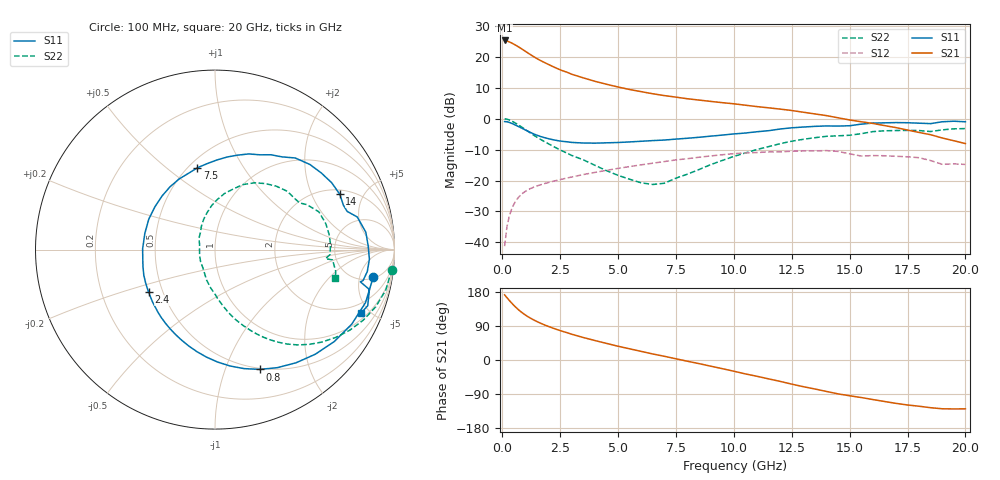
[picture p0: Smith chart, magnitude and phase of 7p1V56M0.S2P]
! Infineon Technologies  Discrete & RF Semiconductors
! bfp620
! VCE =  1.5 V,  IC =  6.0 mA
! Common Emitter S-Parameters:  Sep 2002
# GHz  S  MA  R  50
!  f  S11  S21  S12  S22
! GHz  MAG  ANG  MAG  ANG  MAG  ANG  MAG  ANG
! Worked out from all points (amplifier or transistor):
!   59 points, 100 MHz to 20 GHz, reference 50 ohm
!   highest |S21| = 25.2 dB at 100 MHz (marker M1)
!   |S21| within 3 dB of that: start of sweep to 895 MHz
!   unconditionally stable (mu >= 1): 4.674 GHz to 11.28 GHz; 14.93 GHz to 15.1 GHz; 17.11 GHz to end of sweep
!   at 1 GHz: K = 0.36, MSG = 22.6 dB, |S12| = -23.5 dB
!   at 5.5 GHz: K = 1.04, MAG = 11.2 dB, |S12| = -15.5 dB
!   at 20 GHz: K = 1.39, MAG = -0.3 dB, |S12| = -14.8 dB
!   S11 on the Smith chart (normalised r, x): 100 MHz: 5.35, -8.21; 800 MHz: 0.49, -1.33; 2.4 GHz: 0.42, -0.25; 7.5 GHz: 0.55, +0.65; 14 GHz: 2.24, +3.28; 20 GHz: 1.34, -4.46
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0.1  0.8951 -9.8  18.27 172.0  0.0087 82.1  0.9908 -6.5
0.2  0.8891 -19.4  17.92 164.5  0.0178 80.2  0.9779 -13.3
0.3  0.8678 -28.6  17.35 157.4  0.0264 75.6  0.9505 -19.6
0.4  0.8391 -37.6  16.66 150.6  0.0342 70.9  0.9145 -25.5
0.5  0.8076 -46.2  15.92 144.1  0.0414 66.6  0.874 -31.0
0.6  0.7756 -54.4  15.16 138.2  0.0478 62.8  0.8313 -36.1
0.8  0.713 -69.4  13.64 127.5  0.0586 56.3  0.7453 -45.1
1.1  0.6265 -88.7  11.52 114.6  0.0704 48.9  0.6256 -55.6
1.3  0.5777 -100.0  10.31 107.6  0.0765 45.3  0.557 -61.1
1.5  0.5382 -110.1  9.298 101.4  0.0816 42.5  0.4989 -65.7
1.9  0.4836 -127.9  7.784 90.7  0.0909 38.6  0.4095 -73.3
2.4  0.4399 -147.2  6.36 79.6  0.1014 34.9  0.3256 -81.0
3  0.4122 -166.9  5.203 68.0  0.1139 31.1  0.2537 -89.2
3.5  0.4033 179.5  4.546 59.3  0.1248 28.1  0.2158 -96.3
5  0.4111 144.5  3.237 36.3  0.157 18.5  0.1211 -124.1
7  0.4502 109.0  2.352 9.8  0.2023 4.0  0.0903 161.9
7.5  0.4665 102.1  2.221 3.2  0.215 -0.5  0.1093 144.9
10.5  0.5846 64.6  1.644 -36.7  0.2782 -30.6  0.2786 87.5
13.5  0.749 29.9  1.189 -76.5  0.3009 -62.4  0.4913 46.0
14  0.7607 23.9  1.117 -83.0  0.3042 -68.7  0.5177 38.9
17  0.8619 -3.5  0.715 -114.4  0.2464 -93.1  0.6417 7.4
20  0.8882 -23.3  0.395 -128.9  0.1818 -106.4  0.6896 -13.5
